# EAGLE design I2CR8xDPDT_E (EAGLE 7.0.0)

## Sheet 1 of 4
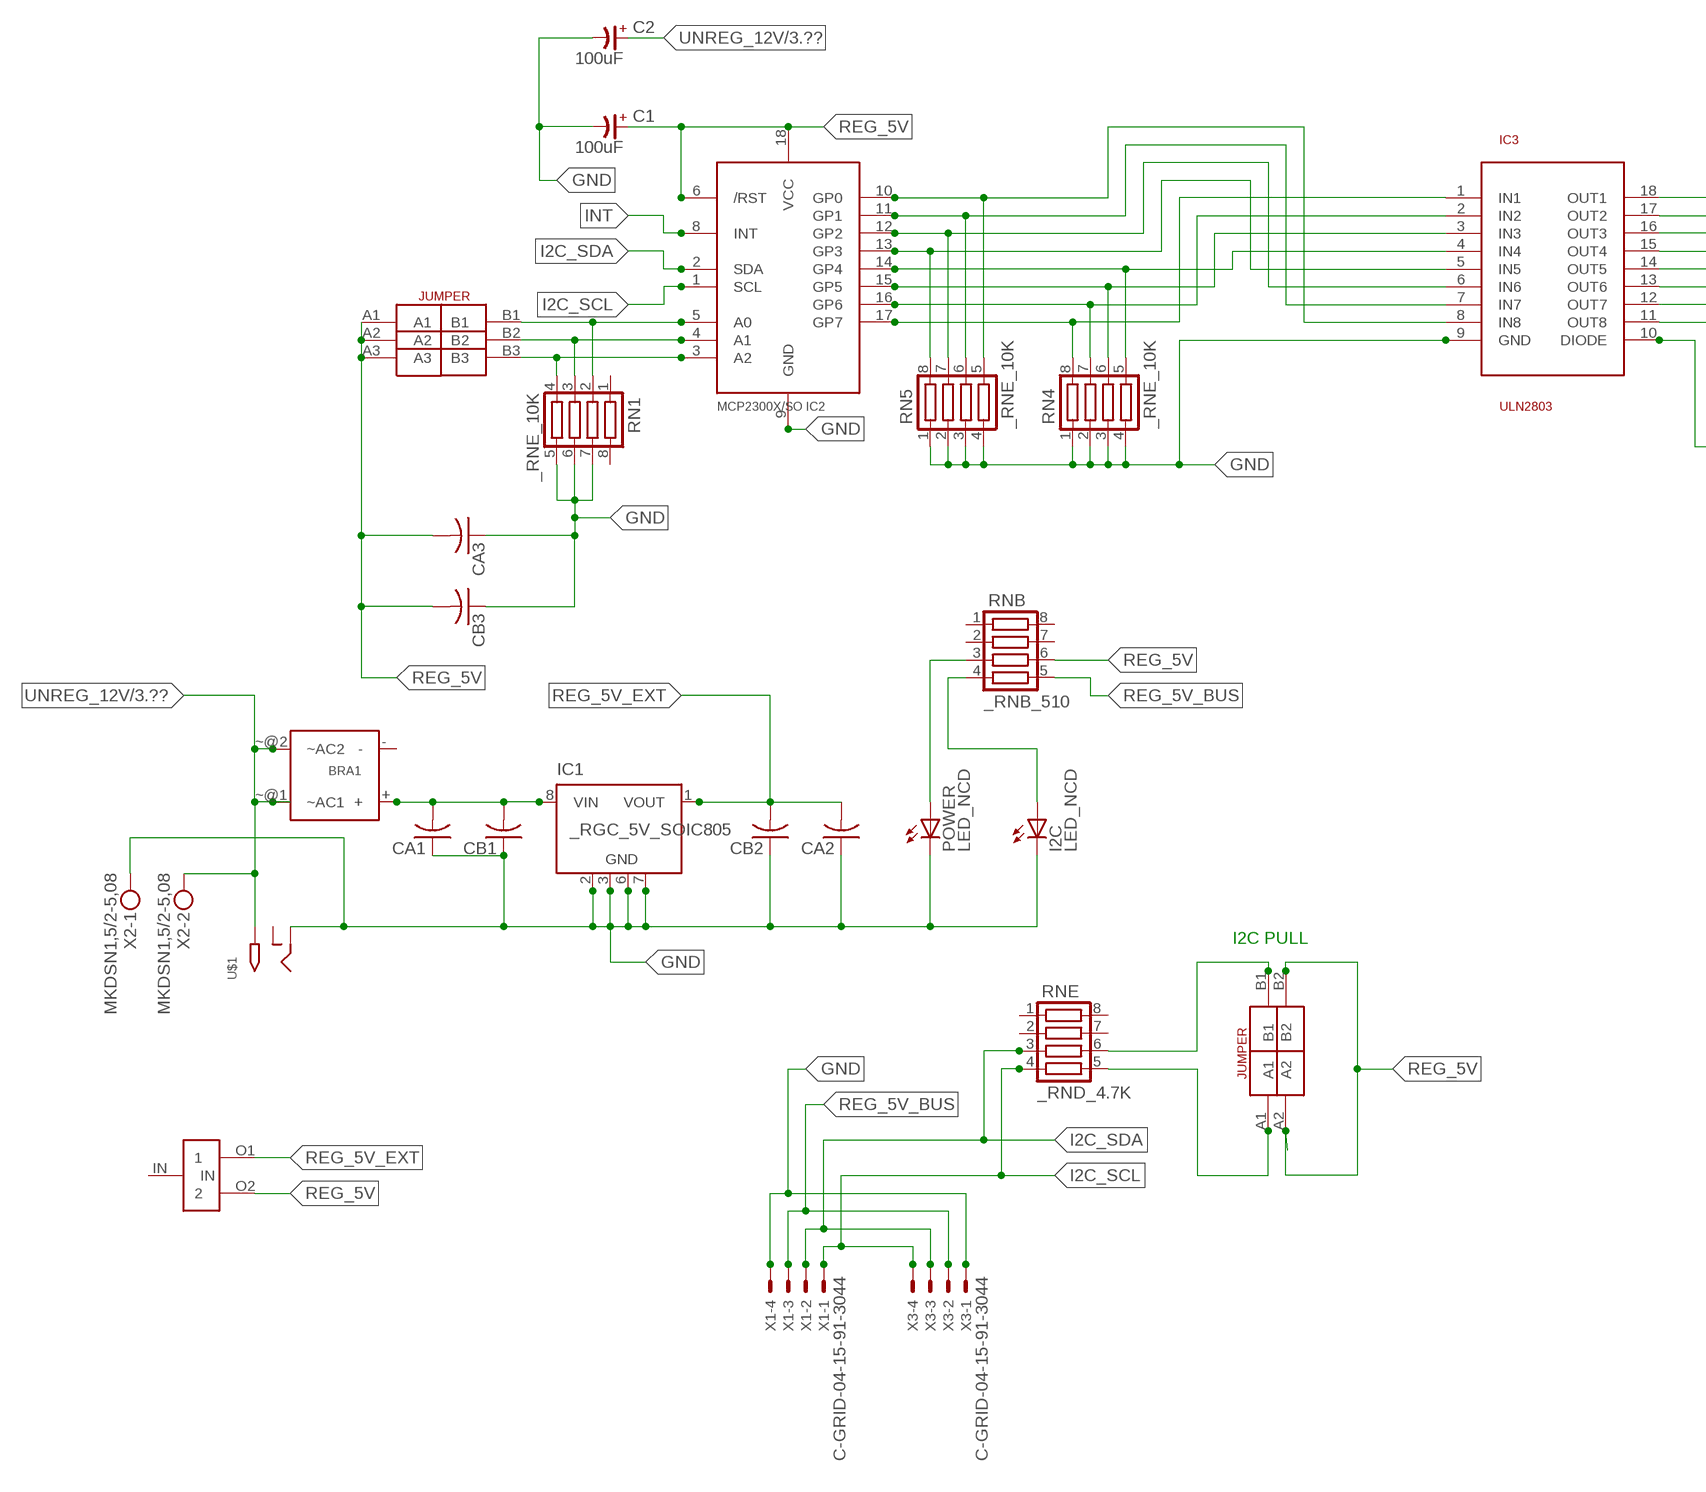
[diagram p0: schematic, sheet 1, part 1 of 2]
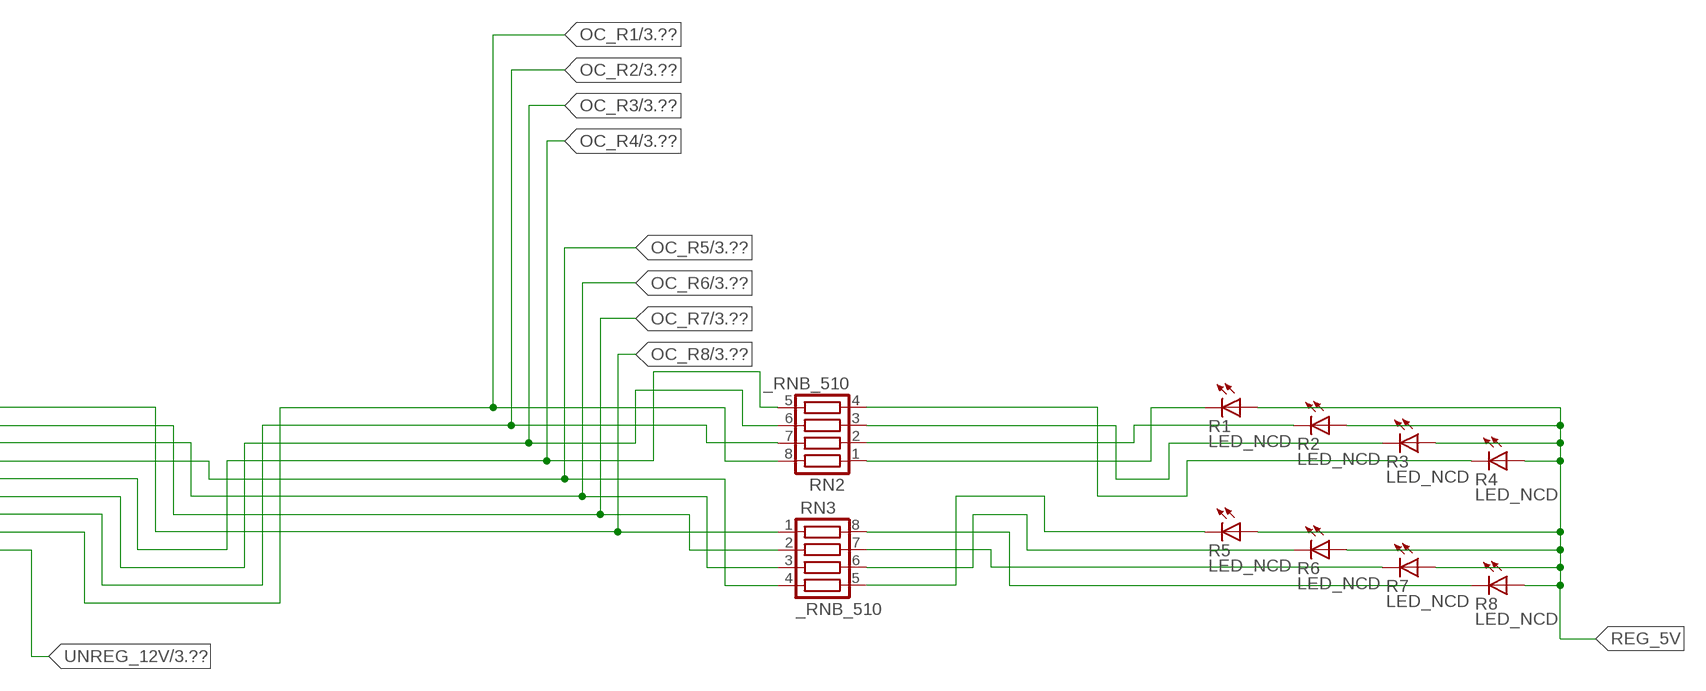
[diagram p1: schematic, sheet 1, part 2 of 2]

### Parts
BRA1  MB2S_  [MB2S]
C1  100uF  CP-E-025X060  [E-025X060]
C2  100uF  CP-E-025X060  [E-025X060]
CA1  CC1206KRX7R9BB104C1206K  [CC1206KRX7R9BB104]
CA2  CC1206KRX7R9BB104C1206K  [CC1206KRX7R9BB104]
CA3  CC1206KRX7R9BB104C1206K  [CC1206KRX7R9BB104]
CB1  TMK316F106ZL-TC1206K  [TMK316F106ZL-T]
CB2  TMK316F106ZL-TC1206K  [TMK316F106ZL-T]
CB3  TMK316F106ZL-TC1206K  [TMK316F106ZL-T]
I2C  LED_NCD  [CHIPLED_0603]
IC1  _RGC_5V_SOIC805  [_RGC_5V_SOIC8]
IC2  MCP2300X/SO  [SO18W]
IC3  ULN2803  [SO18L]
POWER  LED_NCD  [CHIPLED_0603]
R1  LED_NCD  [CHIPLED_0603]
R2  LED_NCD  [CHIPLED_0603]
R3  LED_NCD  [CHIPLED_0603]
R4  LED_NCD  [CHIPLED_0603]
R5  LED_NCD  [CHIPLED_0603]
R6  LED_NCD  [CHIPLED_0603]
R7  LED_NCD  [CHIPLED_0603]
R8  LED_NCD  [CHIPLED_0603]
RN1  _RNE_10K  [RNE]
RN2  _RNB_510  [RNB]
RN3  _RNB_510  [RNB]
RN4  _RNE_10K  [RNE]
RN5  _RNE_10K  [RNE]
RNB  _RNB_510  [RNB]
RNE  _RND_4.7K  [RND]
U$1  2.1MMJACK  [PJ-102A]
U$3  JUMPER_2X2  [JUMPER_2X2]
U$5  LINK_2  [LINK_2]
U$18  JUMPER_3X2  [JUMPER_3X2]
X1  C-GRID-04-15-91-3044  [15-91-04]
X2  MKDSN1,5/2-5,08  [MKDSN1,5/2-5,08]
X3  C-GRID-04-15-91-3044  [15-91-04]

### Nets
GND: C1.- C2.- CA1.1 CA2.1 CA3.1 CB1.1 CB2.1 CB3.1 I2C.C IC1.2(GND) IC1.3(GND) IC1.6(GND) IC1.7(GND) IC2.9(GND) IC3.9(GND) POWER.C RN1.5 RN1.6 RN1.7 RN4.1 RN4.2 RN4.3 RN4.4 RN5.1 RN5.2 RN5.3 RN5.4 U$1.RING X1.4 X2.1 X3.1
GP4: IC2.14(GP4) IC3.4(IN4) RN4.5
GP6: IC2.16(GP6) IC3.2(IN2) RN4.7
I2C_SCL: IC2.1(SCL) RNE.4 X1.1 X3.4
I2C_SDA: IC2.2(SDA) RNE.3 X1.2 X3.3
INT: IC2.8(INT)
N$1: BRA1.+ CA1.2 CB1.2 IC1.8(VIN)
N$2: POWER.A RNB.3
N$3: I2C.A RNB.4
N$4: RNE.5 U$3.A1
N$5: RNE.6 U$3.B1
N$6: IC2.5(A0) RN1.2 U$18.B1
N$7: IC2.4(A1) RN1.3 U$18.B2
N$8: IC2.3(A2) RN1.4 U$18.B3
N$20: R1.C RN2.1
N$21: IC2.12(GP2) IC3.6(IN6) RN5.7
N$22: IC2.11(GP1) IC3.7(IN7) RN5.6
N$23: IC2.10(GP0) IC3.8(IN8) RN5.5
N$29: R2.C RN2.2
N$30: R3.C RN2.3
N$31: R4.C RN2.4
N$32: R8.C RN3.8
N$81: R7.C RN3.7
N$82: R6.C RN3.6
N$83: R5.C RN3.5
N$89: IC2.13(GP3) IC3.5(IN5) RN5.8
N$93: IC2.15(GP5) IC3.3(IN3) RN4.6
N$94: IC2.17(GP7) IC3.1(IN1) RN4.8
OC_R1: IC3.11(OUT8) RN2.8 ; also sheet 3
OC_R2: IC3.12(OUT7) RN2.7 ; also sheet 3
OC_R3: IC3.13(OUT6) RN2.6 ; also sheet 3
OC_R4: IC3.14(OUT5) RN2.5 ; also sheet 3
OC_R5: IC3.15(OUT4) RN3.4 ; also sheet 3
OC_R6: IC3.16(OUT3) RN3.3 ; also sheet 3
OC_R7: IC3.17(OUT2) RN3.2 ; also sheet 3
OC_R8: IC3.18(OUT1) RN3.1 ; also sheet 3
REG_5V: C1.+ CA3.2 CB3.2 IC2.6(/RST) IC2.18(VCC) R1.A R2.A R3.A R4.A R5.A R6.A R7.A R8.A RNB.6 U$3.A2 U$3.B2 U$5.O2 U$18.A1 U$18.A2 U$18.A3
REG_5V_BUS: RNB.5 X1.3 X3.2
REG_5V_EXT: CA2.2 CB2.2 IC1.1(VOUT) U$5.O1
UNREG_12V: BRA1.~@1(~AC1) BRA1.~@2(~AC2) C2.+ IC3.10(DIODE) U$1.TIP X2.2 ; also sheet 3
Unconnected: BRA1.- IC1.4(NC) IC1.5(NC) RN1.1 RN1.8 RNB.1 RNB.2 RNB.7 RNB.8 RNE.1 RNE.2 RNE.7 RNE.8 U$1.RING_SW U$5.IN

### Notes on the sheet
- I2C PULL

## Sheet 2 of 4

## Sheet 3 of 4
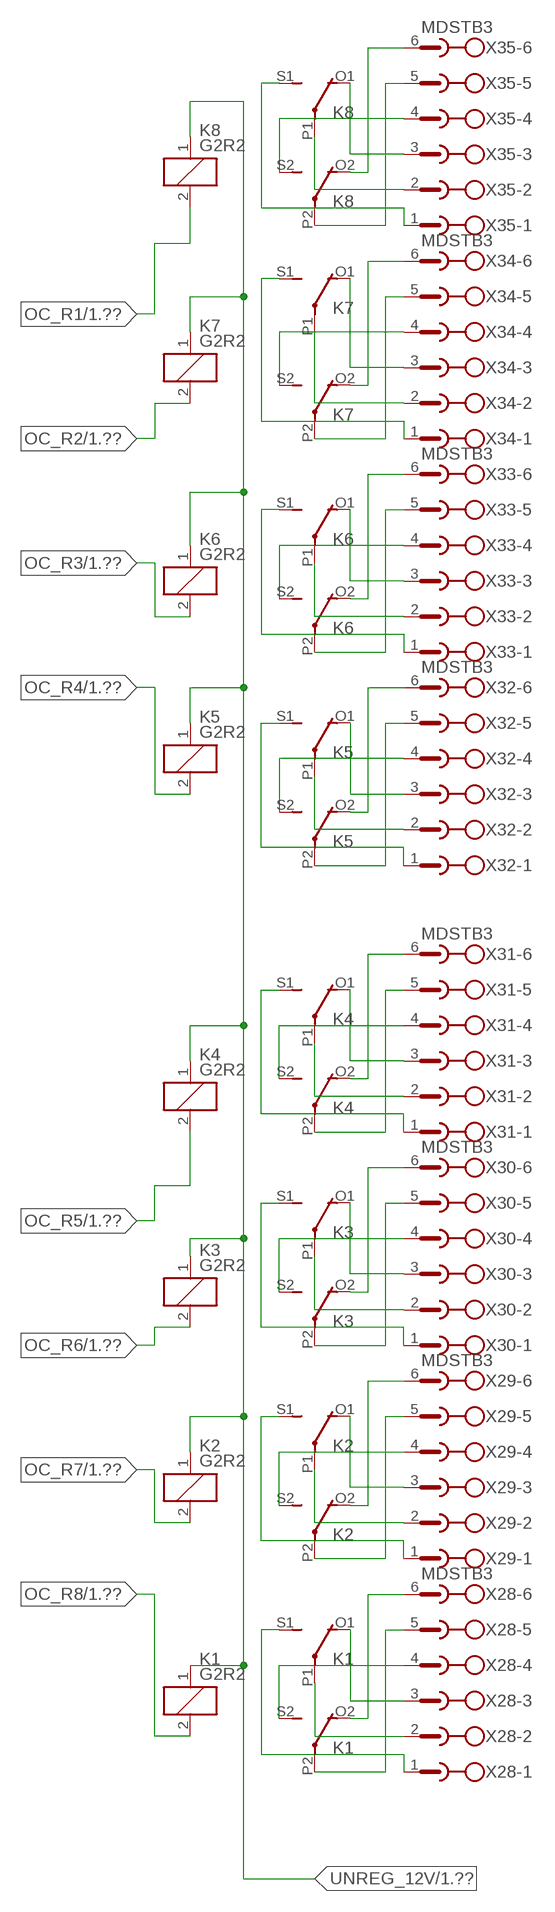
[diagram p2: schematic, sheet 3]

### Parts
K1  G2R2  [G2R2]
K2  G2R2  [G2R2]
K3  G2R2  [G2R2]
K4  G2R2  [G2R2]
K5  G2R2  [G2R2]
K6  G2R2  [G2R2]
K7  G2R2  [G2R2]
K8  G2R2  [G2R2]
X28  MDSTB3  [MDSTB3]
X29  MDSTB3  [MDSTB3]
X30  MDSTB3  [MDSTB3]
X31  MDSTB3  [MDSTB3]
X32  MDSTB3  [MDSTB3]
X33  MDSTB3  [MDSTB3]
X34  MDSTB3  [MDSTB3]
X35  MDSTB3  [MDSTB3]

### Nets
N$84: K1.P2(3:COM) X28.5
N$85: K1.O2(3:NC) X28.6
N$86: K1.S2(3:NO) X28.4
N$87: K1.P1(2:COM) X28.2
N$88: K1.O1(2:NC) X28.3
N$90: K1.S1(2:NO) X28.1
N$91: K2.P2(3:COM) X29.5
N$92: K2.O2(3:NC) X29.6
N$95: K2.S2(3:NO) X29.4
N$96: K2.S1(2:NO) X29.1
N$97: K2.P1(2:COM) X29.2
N$98: K2.O1(2:NC) X29.3
N$99: K3.P2(3:COM) X30.5
N$100: K3.O2(3:NC) X30.6
N$101: K4.P2(3:COM) X31.5
N$102: K4.O2(3:NC) X31.6
N$103: K3.S2(3:NO) X30.4
N$104: K4.S2(3:NO) X31.4
N$105: K3.O1(2:NC) X30.3
N$106: K4.O1(2:NC) X31.3
N$107: K4.P1(2:COM) X31.2
N$108: K3.P1(2:COM) X30.2
N$109: K3.S1(2:NO) X30.1
N$110: K4.S1(2:NO) X31.1
N$111: K5.O2(3:NC) X32.6
N$112: K5.P2(3:COM) X32.5
N$113: K5.S2(3:NO) X32.4
N$114: K5.P1(2:COM) X32.2
N$115: K5.S1(2:NO) X32.1
N$116: K5.O1(2:NC) X32.3
N$117: K6.P2(3:COM) X33.5
N$118: K6.O2(3:NC) X33.6
N$119: K6.P1(2:COM) X33.2
N$120: K6.S1(2:NO) X33.1
N$121: K7.P1(2:COM) X34.2
N$122: K8.P1(2:COM) X35.2
N$316: K8.P2(3:COM) X35.5
N$317: K8.O2(3:NC) X35.6
N$318: K6.O1(2:NC) X33.3
N$319: K8.O1(2:NC) X35.3
N$320: K7.O1(2:NC) X34.3
N$321: K7.O2(3:NC) X34.6
N$322: K7.P2(3:COM) X34.5
N$323: K6.S2(3:NO) X33.4
N$324: K7.S2(3:NO) X34.4
N$325: K7.S1(2:NO) X34.1
N$326: K8.S1(2:NO) X35.1
N$327: K8.S2(3:NO) X35.4
OC_R1: K8.2(1:C2) ; also sheet 1
OC_R2: K7.2(1:C2) ; also sheet 1
OC_R3: K6.2(1:C2) ; also sheet 1
OC_R4: K5.2(1:C2) ; also sheet 1
OC_R5: K4.2(1:C2) ; also sheet 1
OC_R6: K3.2(1:C2) ; also sheet 1
OC_R7: K2.2(1:C2) ; also sheet 1
OC_R8: K1.2(1:C2) ; also sheet 1
UNREG_12V: K1.1(1:C1) K2.1(1:C1) K3.1(1:C1) K4.1(1:C1) K5.1(1:C1) K6.1(1:C1) K7.1(1:C1) K8.1(1:C1) ; also sheet 1

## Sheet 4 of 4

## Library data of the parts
BRA1 = NCD_ULTIMATE_LIBRARY:MB2S: Bridge Rectifier BRA MB2S 200V 500ma Digikey MB2S-TPMSTR-ND/MB2S-TP
C1 C2 = NCD_ULTIMATE_LIBRARY:CP-: Capacitors All Kinds POLARIZED CAP
CA1-CA3 = NCD_ULTIMATE_LIBRARY:CC1206KRX7R9BB104: Capacitor CA .1uF 50V SMT C1206K CC1206KRX7R9BB104
CB1-CB3 = NCD_ULTIMATE_LIBRARY:TMK316F106ZL-T: Capacitor CB 10uF SMT 1206 TMK316F106ZL-T
I2C POWER = NCD_ULTIMATE_bhaskar:LED_NCD
IC1 = NCD_ULTIMATE_LIBRARY:_RGC_5V_SOIC8: Regulator Linear 5V Chip Positive VOLTAGE REGULATOR Digikey 497-7267-2-ND/L78L05CD13TR
IC2 = NCD_ULTIMATE_LIBRARY:MCP2300X: Semiconductor Port Expander I/O 8-Bit I2C MCP23008 Inexpensive i2c i/o expander - 8 general purpose i/o pins with optional pullups
IC3 = NCD_ULTIMATE_LIBRARY:ULN2803: Semiconductor 8 O.C. N-Channel Transistor Driver Digikey ULN2803AFWGCELTR-ND/ULN2803AFWG,C,EL
K1-K8 = NCD_ULTIMATE_LIBRARY:G2R2: RELAY 2 x switch, Omron
R1-R8 = NCD_ULTIMATE_LIBRARY:LED_NCD: LED Digikey 754-1132-2-ND/APT2012SRCPRV
RN1 RN4 RN5 = NCD_ULTIMATE_LIBRARY:_RNE_10K: Resistor Array RNE SMT 10K x 4 Single Resistor Source: http://www.ctscorp.com/components/Datasheets/CTSChipArrayDs.pdf Digikey 742C083103JPTR-ND/742C083103JP; OC_FARNELL: unknown; OC_NEWARK: unknown
RN2 RN3 RNB = NCD_ULTIMATE_LIBRARY:_RNB_510: Resistor Array RNB SMT 510 x 4 Single Resistor Source: http://www.ctscorp.com/components/Datasheets/CTSChipArrayDs.pdf Digikey 742C083511JPTR-ND/ 742C083511JP; OC_FARNELL: unknown; OC_NEWARK: unknown
RNE = NCD_ULTIMATE_LIBRARY:_RND_4.7K: Resistor Array RND SMT 4.7K x 4 Single Resistor Source: http://www.ctscorp.com/components/Datasheets/CTSChipArrayDs.pdf Digikey 742C083472JPTR-ND/742C083472JP; OC_FARNELL: unknown; OC_NEWARK: unknown
U$1 = NCD_ULTIMATE_CONNECTORS:2.1MMJACK: 2.1mm x 5.5mm DC jack with internal switch. Digikey part #PJ-102A, 4UCON part #05537 By microbuilder.eu
U$3 = NCD_ULTIMATE_CONNECTORS:JUMPER_2X2
U$5 = NCD_ULTIMATE_LIBRARY:LINK_2: PAD_top
U$18 = NCD_ULTIMATE_CONNECTORS:JUMPER_3X2
X1 X3 = NCD_ULTIMATE_CONNECTORS:C-GRID-04: CONNECTOR 4-Pos I2C wire to board 2.54 mm (0.100") pitch header Digikey WM1342-ND/0015912045; OC_FARNELL: unknown; OC_NEWARK: unknown
X2 = NCD_ULTIMATE_CONNECTORS:MKDSN1,5/2-5,08: MKDSN 1,5/ 2-5,08 Printklemme
X28-X35 = NCD_ULTIMATE_LIBRARY:MDSTB3: PHOENIX

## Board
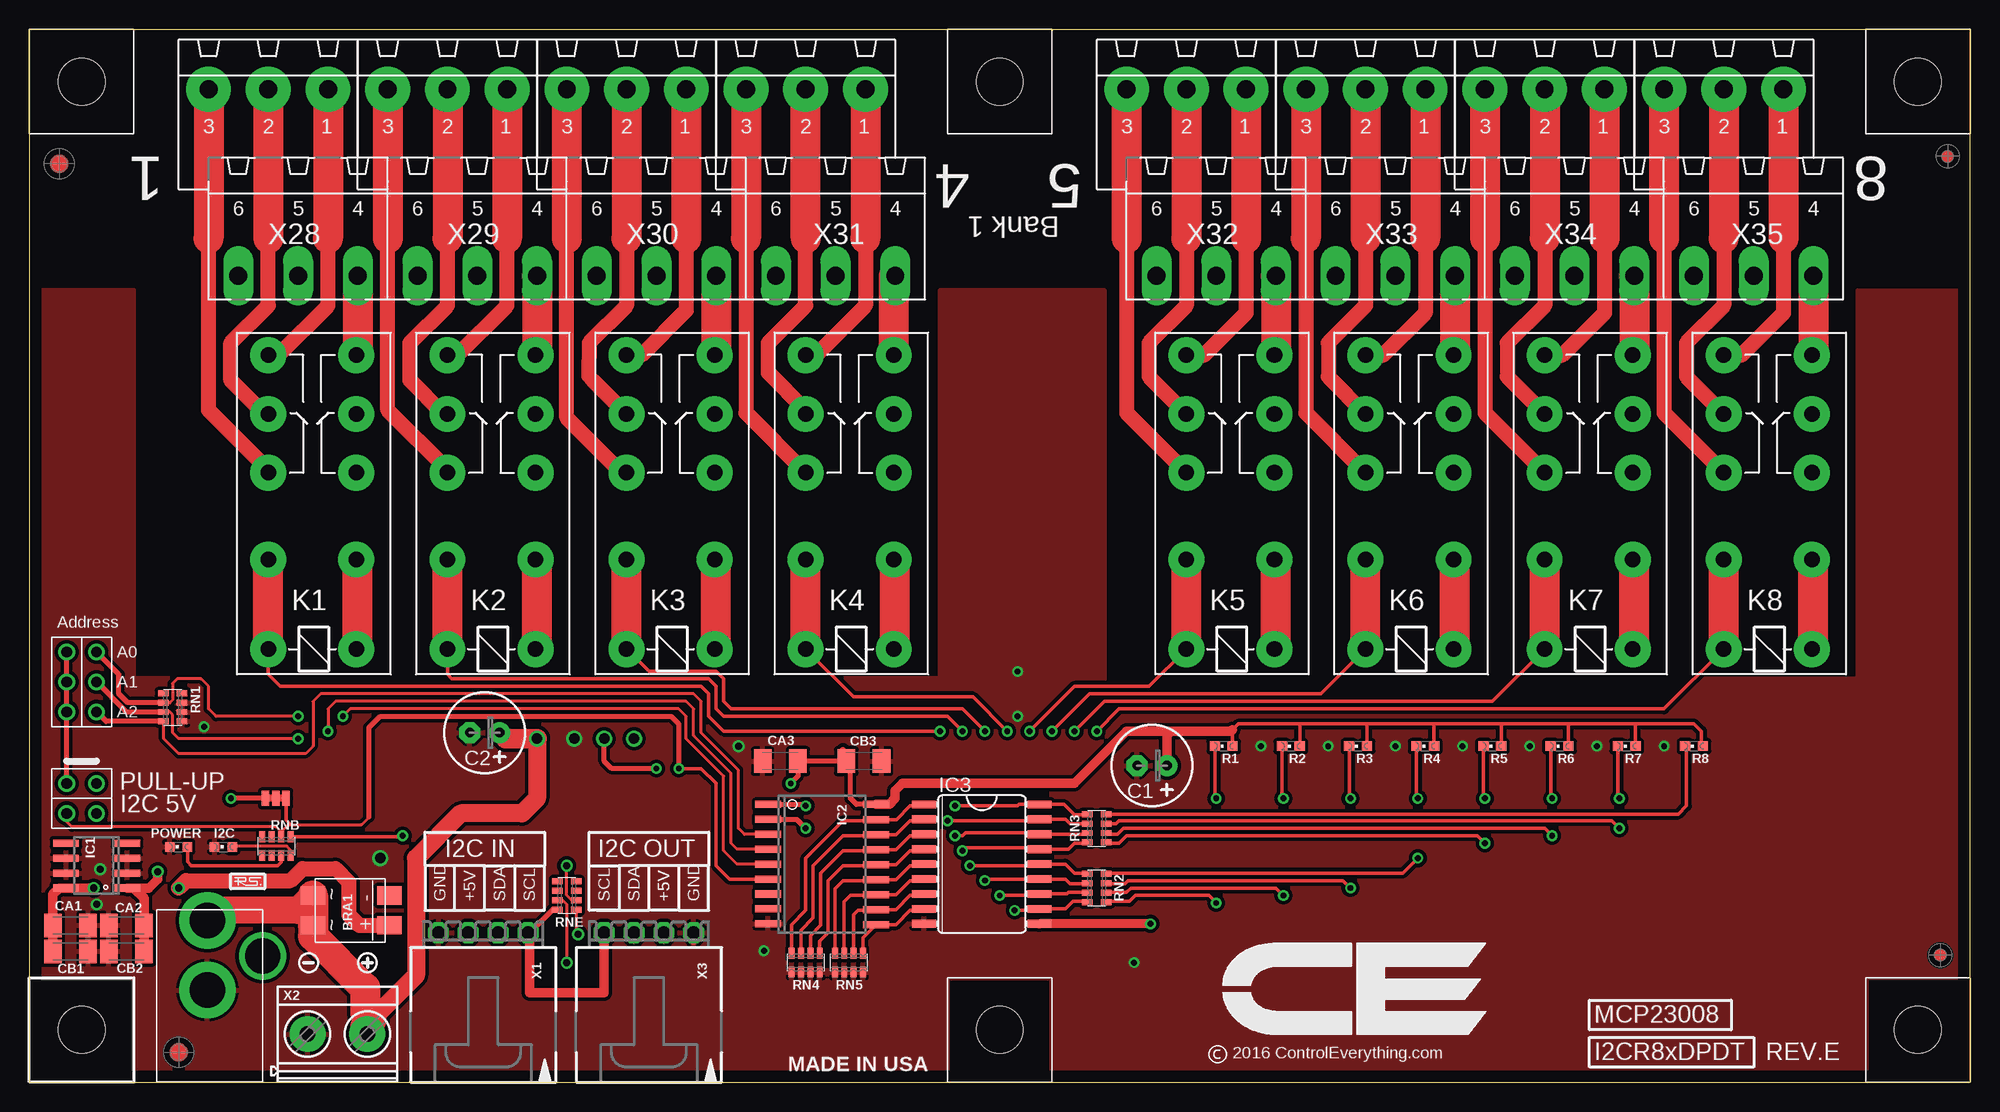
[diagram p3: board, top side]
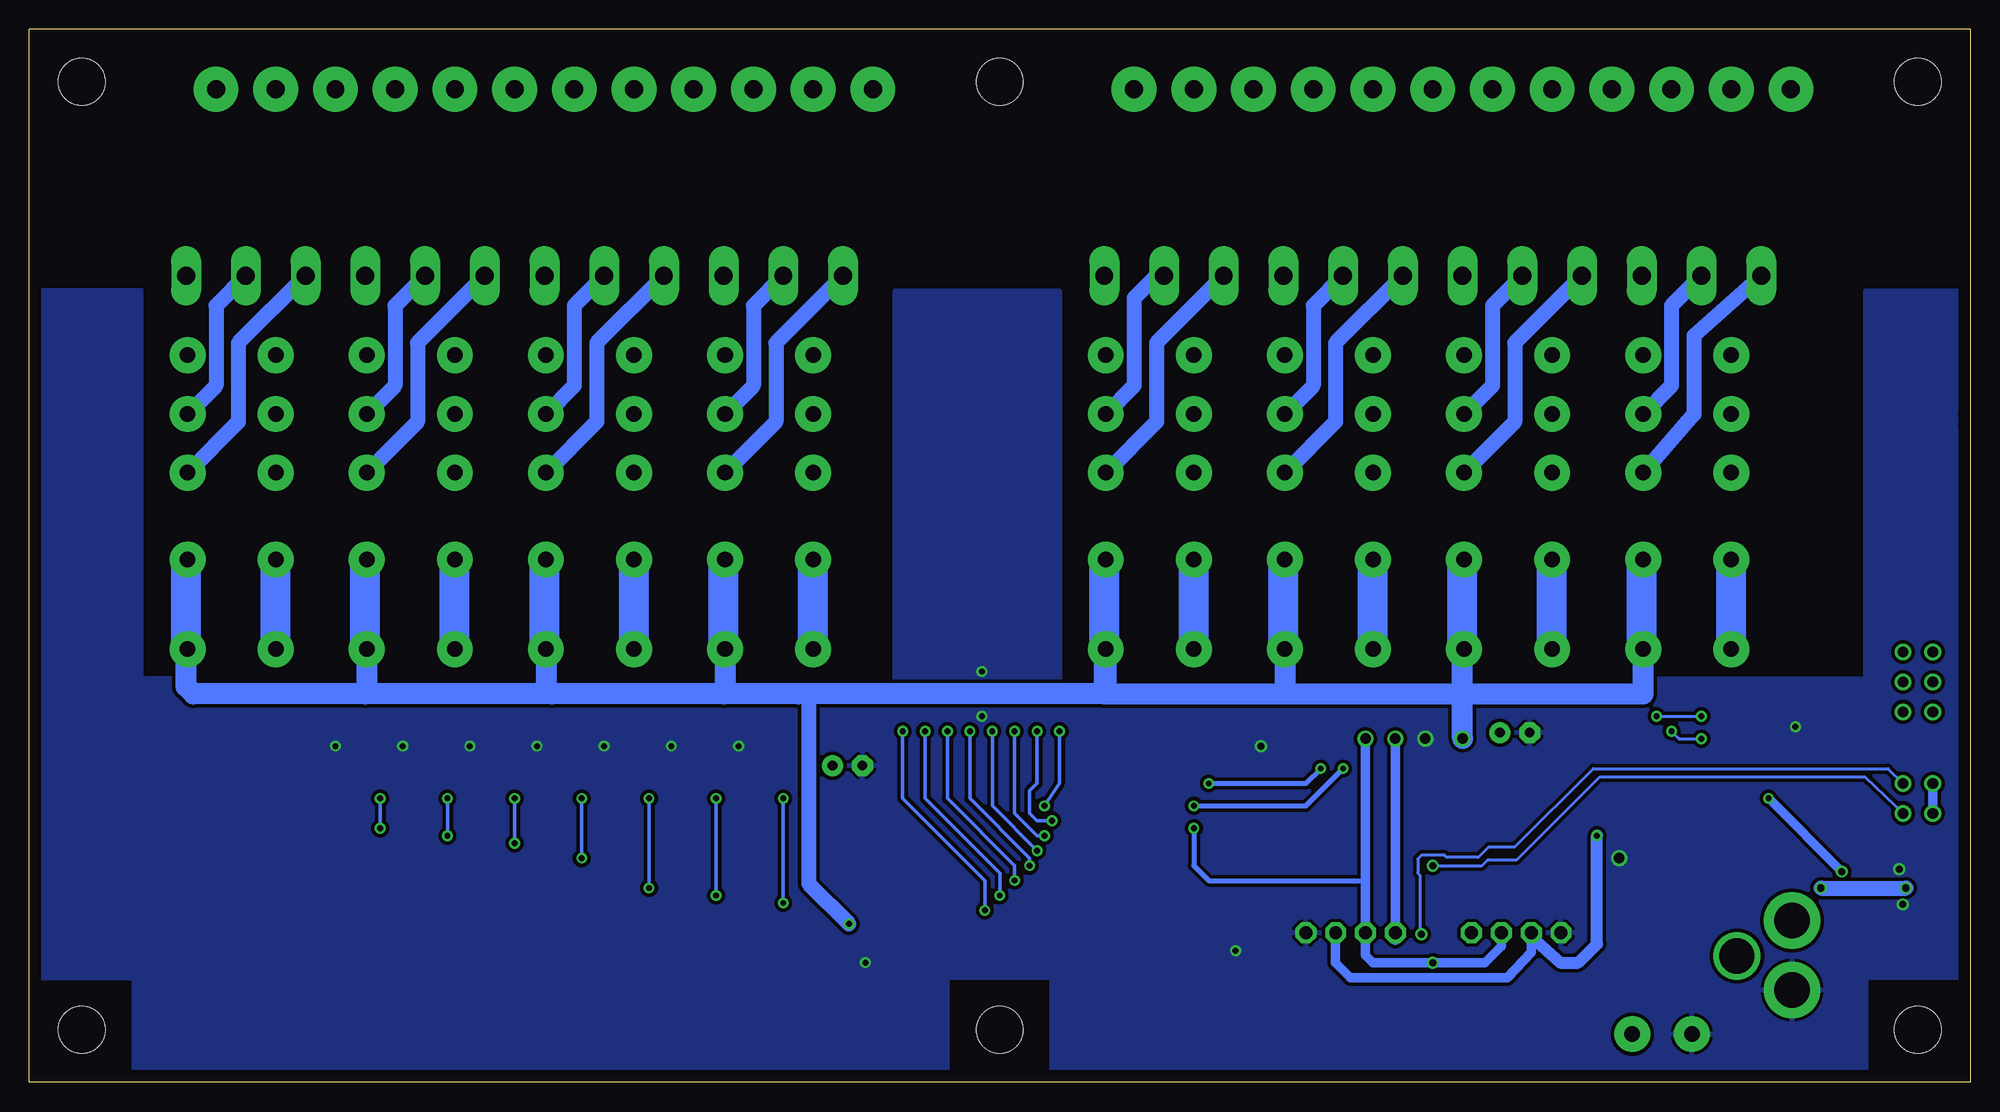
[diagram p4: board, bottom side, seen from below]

Size 165.1 x 89.53 mm. Coordinates in mm from the lower left corner, seen from the top.
Outline: 81.28,0 0,0 0,55.88
Outline: 81.28,0 82.53,0
Outline: 0,56.82 0,55.88
Outline: 81.28,0 165.1,0 165.1,89.53 0,89.53 0,55.88
Copper layers (1*16): Top 0.035mm / dielectric 1.5mm / Bottom 0.035mm
Design rules "default": minimum track width 10mil, minimum drill 24mil, track to track 8mil, track to pad 8mil, pad to pad 8mil, via to via 8mil, smd to smd 8mil, copper to edge 40mil, drill to drill 8mil, minimum pad ring 10mil, minimum via ring 8mil, stop-mask expansion 4mil, vias tented up to drill 0mil, thermal gap 10mil
Holes 3.96 mm at 4.45,4.45

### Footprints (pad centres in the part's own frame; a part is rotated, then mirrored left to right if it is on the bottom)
MB2S = smd 1.55 x 2.1: + 0,-6.5; - 2.54,-6.5; ~@1 0,0; ~@2 2.54,0
E-025X060 = drill 0.813 pad 1.778: + -1.27,0 | drill 0.813 pad 1.778 octagon: - 1.27,0
CC1206KRX7R9BB104 = smd 1.5 x 2: 1 -1.5,0; 2 1.5,0
TMK316F106ZL-T = smd 1.5 x 2: 1 -1.5,0; 2 1.5,0
CHIPLED_0603 = smd 0.8 x 0.8: A 0,-0.75; C 0,0.75
_RGC_5V_SOIC8 = smd 0.6 x 2.2: 1 -1.905,-2.6; 2 -0.635,-2.6; 3 0.635,-2.6; 4 1.905,-2.6; 5 1.905,2.6; 6 0.635,2.6; 7 -0.635,2.6; 8 -1.905,2.6
SO18W = smd 0.6 x 2.2: 1 -4.445,-4.6; 2 -3.175,-4.6; 3 -1.905,-4.6; 4 -0.635,-4.6; 5 0.635,-4.6; 6 1.905,-4.6; 7 3.175,-4.6; 8 4.445,-4.6; 9 5.715,-4.6; 10 5.775,4.6; 11 4.505,4.6; 12 3.235,4.6; 13 1.965,4.6; 14 0.695,4.6; 15 -0.575,4.6; 16 -1.845,4.6; 17 -3.145,4.6; 18 -4.445,4.6
SO18L = smd 0.66 x 2.032: 1 -5.08,-4.902; 2 -3.81,-4.902; 3 -2.54,-4.902; 4 -1.27,-4.902; 5 0,-4.902; 6 1.27,-4.902; 7 2.54,-4.902; 8 3.81,-4.902; 9 5.08,-4.902; 10 5.08,4.902; 11 3.81,4.902; 12 2.54,4.902; 13 1.27,4.902; 14 0,4.902; 15 -1.27,4.902; 16 -2.54,4.902; 17 -3.81,4.902; 18 -5.08,4.902
G2R2 = drill 1.321 pad 3.048: 1 -2.54,-3.683; 2 -2.54,3.81; 3 5.08,-3.683; 4 5.08,3.81; O1 12.471,3.81; O2 12.471,-3.683; P1 17.45,3.81; P2 17.45,-3.683; S1 22.454,3.81; S2 22.454,-3.683
CHIPLED_0603' = smd 0.8 x 0.876: A 0,-0.75; C 0,0.75
RNE = smd 0.5 x 0.9: 1 -1.2,-0.8; 2 -0.4,-0.8; 3 0.4,-0.8; 4 1.2,-0.8; 5 1.2,0.8; 6 0.4,0.8; 7 -0.4,0.8; 8 -1.2,0.8
RNB = smd 0.5 x 0.9: 1 -1.2,-0.8; 2 -0.4,-0.8; 3 0.4,-0.8; 4 1.2,-0.8; 5 1.2,0.8; 6 0.4,0.8; 7 -0.4,0.8; 8 -1.2,0.8
RND = smd 0.5 x 0.9: 1 -1.2,-0.8; 2 -0.4,-0.8; 3 0.4,-0.8; 4 1.2,-0.8; 5 1.2,0.8; 6 0.4,0.8; 7 -0.4,0.8; 8 -1.2,0.8
PJ-102A = drill 3 pad 4.8: RING 0.1,-3.39; TIP 0.1,-9.29 | drill 3 pad 3.251: RING_SW -4.6,-6.29
JUMPER_2X2 = drill 0.9: A1 0,2.54; A2 0,0; B1 2.54,2.54; B2 2.54,0
LINK_2 = smd 1.27 x 0.635: IN 0,0; O1 0,0.889; O2 0,-0.889
PCB_MOUNTING_HOLE = hole 3.962: 4.445,4.445
JUMPER_3X2 = drill 0.9: A1 0,5.08; A2 0,2.54; A3 0,0; B1 2.54,5.08; B2 2.54,2.54; B3 2.54,0
15-91-04 = drill 1.1 pad 1.778 octagon: 1 -3.81,-7.62; 2 -1.27,-7.62; 3 1.27,-7.62; 4 3.81,-7.62
MKDSN1,5/2-5,08 = drill 1.3 pad 3.048: 1 -2.561,0.025; 2 2.519,0.025
MDSTB3 = drill 1.524 pad 3.81: 1 -3.81,-10.795; 2 1.27,-10.795; 3 6.35,-10.795 | drill 1.524 pad 2.54 long: 4 -6.35,5.08; 5 -1.27,5.08; 6 3.81,5.08

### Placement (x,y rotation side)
BRA1  24.13,13.34 90 top
C1  95.5,26.92 180 top
C2  38.73,29.72 180 top
CA1  3.49,13.34 180 top
CA2  8.26,13.34 0 top
CA3  63.88,27.3 0 top
CB1  3.49,11.11 180 top
CB2  8.26,11.11 0 top
CB3  70.99,27.3 180 top
I2C  16.51,20 90 top
IC1  5.71,18.41 90 top
IC2  67.44,19.18 270 top
IC3  81.03,18.54 270 top
K1  24.13,39.37 90 top
K2  39.37,39.37 90 top
K3  54.61,39.37 90 top
K4  69.85,39.37 90 top
K5  102.23,39.37 90 top
K6  117.47,39.37 90 top
K7  132.72,39.37 90 top
K8  147.96,39.37 90 top
POWER  12.7,20 90 top
R1  LED_NCD  [CHIPLED_0603']  101.6,28.57 90 top
R2  LED_NCD  [CHIPLED_0603']  107.31,28.57 90 top
R3  LED_NCD  [CHIPLED_0603']  113.03,28.57 90 top
R4  LED_NCD  [CHIPLED_0603']  118.75,28.57 90 top
R5  LED_NCD  [CHIPLED_0603']  124.46,28.57 90 top
R6  LED_NCD  [CHIPLED_0603']  130.18,28.57 90 top
R7  LED_NCD  [CHIPLED_0603']  135.89,28.57 90 top
R8  LED_NCD  [CHIPLED_0603']  141.6,28.57 90 top
RN1  12.19,31.88 270 top
RN2  90.81,16.51 90 top
RN3  90.81,21.59 270 top
RN4  66.04,10.16 0 top
RN5  69.72,10.16 0 top
RNB  21.02,20.07 0 top
RNE  45.72,15.88 270 top
U$1  15.24,4.45 180 top
U$3  3.17,25.4 270 top
U$4  [VISION_REF10]  162.56,10.79 270 top
U$5  20.95,24.13 90 top
U$6  PCB_MOUNTING_HOLE  [PCB_MOUNTING_HOLE]  87,0 90 top
U$9  PCB_MOUNTING_HOLE  [PCB_MOUNTING_HOLE]  87,80.64 90 top
U$10  [VISION_REF15]  12.7,2.54 0 top
U$11  PCB_MOUNTING_HOLE  [PCB_MOUNTING_HOLE]  165.1,0 90 top
U$13  PCB_MOUNTING_HOLE  [PCB_MOUNTING_HOLE]  8.89,80.64 90 top
U$14  PCB_MOUNTING_HOLE  [PCB_MOUNTING_HOLE]  165.1,80.64 90 top
U$16  [VISION_REF10]  163.19,78.74 270 top
U$17  [VISION_REF15]  2.54,78.11 270 top
U$18  3.17,31.5 0 top
U$21  [ICON_USA]  64.52,0.89 0 top
U$22  [ICON_MINUS]  23.75,10.16 180 top
U$24  [ICON_PLUS]  28.77,10.16 90 top
X1  38.61,5.08 180 top
X2  26.23,4.06 0 top
X3  52.7,5.08 180 top
X28  21.59,73.66 180 top
X29  36.83,73.66 180 top
X30  52.07,73.66 180 top
X31  67.31,73.66 180 top
X32  99.69,73.66 180 top
X33  114.94,73.66 180 top
X34  130.18,73.66 180 top
X35  145.41,73.66 180 top

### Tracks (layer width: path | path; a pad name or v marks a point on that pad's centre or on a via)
GND  (via drill 0.5, 0.6, 0.9)
  Top 0.406: 34.8,12.38 X1.4
  Top 0.813: X3.1 56.52,12.06
  other vias: 5.71,15.11 6.03,18.1 46.35,29.21 29.84,19.05 14.86,30.23 62.48,11.18 127.64,28.57 93.98,10.16 133.35,28.57 139.06,28.57 121.92,28.57 116.2,28.57 110.49,28.57 104.78,28.57 60.33,28.57 84.07,31.11 84.07,34.92
  pour Bottom (isolate 0.305): 0.64,8.89 8.89,8.89 8.89,0 78.11,0 78.11,8.89 91.44,8.89 91.44,67.31 77.47,67.31 77.47,34.29 8.89,34.29 8.89,67.31 0.64,67.31
  pour Top (isolate 0.305): -1.27,8.89 8.89,8.89 8.89,0 78.11,0 78.11,8.89 91.44,8.89 91.44,67.31 77.47,67.31 77.47,34.29 8.89,34.29 8.89,67.31 -1.27,67.31
  pour Top (isolate 0.305): 87,34.29 155.57,34.29 155.57,67.31 164.47,67.31 164.47,8.89 156.21,8.89 156.21,0 87,0
  pour Bottom (isolate 0.305): 87,0 87,34.29 155.57,34.29 155.57,67.31 164.47,67.31 164.47,8.89 156.21,8.89 156.21,0
GP4
  Top 0.305: RN4.5 67.24,11.99 67.94,12.7 67.94,17.14 69.22,18.41 71.97,18.41 IC2.14 73.73,18.48 74.93,19.68 76,19.68 IC3.4
GP6
  Top 0.305: RN4.7 65.64,12.94 66.67,13.97 66.67,18.41 69.22,20.95 71.97,20.95 IC2.16 73.73,21.02 74.93,22.23 76,22.23 IC3.2
I2C_SCL  (via drill 0.5, 0.9)
  Top 0.406: RNE.4 44.51,14.68 42.55,12.7 | IC2.1 65.91,23.62 v66.04,23.5 | v53.34,26.67 49.53,26.67 48.9,27.3 v48.9,29.21
  Top 0.813: X3.4 48.9,7.62 42.55,7.62 42.55,12.7 X1.1
  Bottom 0.406: v66.04,23.5 56.52,23.5 v53.34,26.67
  Bottom 0.813: v48.9,29.21 X3.4 48.9,12.06
I2C_SDA  (via drill 0.5, 0.6, 0.9)
  Top 0.254: RNE.3 45.36,15.47 45.72,15.11 v45.72,10.16
  Top 0.406: IC2.2 65.28,22.35 v66.04,21.59
  Top 0.61: X3.3 51.44,12.06 | X1.2 39.88,12.38
  Bottom 0.406: v66.04,21.59 66.04,18.41 64.77,17.14 51.44,17.14 | 39.88,12.38 X1.2
  Bottom 0.813: 39.88,12.38 39.88,11.56 41.27,10.16 v45.72,10.16 50.8,10.16 51.44,10.79 X3.3 51.44,17.14 v51.44,29.21
N$1  (via drill 0.6)
  Top 0.813: CB1.2 CA1.2 1.99,15.96 2.54,16.51 IC1.8 v5.46,16.51
  Top 1.27: v12.7,16.51 13.34,17.14 22.23,17.14 23.24,18.16 26.04,18.16 27.18,17.02 27.18,14.22 28.07,13.34 BRA1.+
  Bottom 1.27: v12.7,16.51 v5.46,16.51
N$2
  Top 0.305: RNB.3 21.4,18.95 21.4,18.7 21.12,18.41 13.78,18.41 13.45,18.74 POWER.A
N$3
  Top 0.254: 22.23,18.95 22.23,19.74 21.9,20.07 16.94,20.07
  Top 0.305: RNB.4 22.23,18.95 | 16.94,20.07 I2C.A
N$4  (via drill 0.6)
  Top 0.254: RNE.5 46.52,12.6 v46.67,12.57
  Bottom 0.254: U$3.A1 6.99,26.67 32.07,26.67 38.73,20 40.96,20 41.85,19.11 44.51,19.11 44.7,19.3 46.67,19.3 46.99,18.99 46.99,17.78 46.8,17.59 46.8,12.7 v46.67,12.57
N$5  (via drill 0.6)
  Top 0.254: RNE.6 46.12,15.47 45.72,15.88 v45.72,18.41
  Bottom 0.254: v45.72,18.41 41.53,18.41 41.02,18.92 38.54,18.92 31.5,25.97 8.95,25.97 6.35,23.5 U$3.B1
N$6  (via drill 0.5)
  Top 0.254: IC2.5 60.2,18.54 59.05,19.68 59.05,26.04 55.88,29.21 55.88,31.11 55.24,31.75 27.3,31.75 v26.67,31.11 | v22.86,31.11 15.88,31.11 15.24,31.75 15.24,33.66 14.61,34.29 12.57,34.29 12.19,33.91 12.19,32.51 11.94,32.26 11.41,32.26 RN1.2
  Top 0.406: RN1.2 8.36,32.28 7.62,33.02 7.62,34.67 U$18.B1
  Bottom 0.254: v26.67,31.11 v22.86,31.11
N$7  (via drill 0.5)
  Top 0.254: IC2.4 60.2,19.81 59.69,20.32 59.69,26.29 56.52,29.46 56.52,31.75 55.88,32.38 26.04,32.38 25.4,31.75 v25.4,29.84 | v22.86,29.21 12.7,29.21 12.19,29.72 12.19,31.24 11.94,31.5 11.41,31.5 RN1.3
  Top 0.406: RN1.3 8.27,31.48 U$18.B2
  Bottom 0.254: v25.4,29.84 24.77,29.21 v22.86,29.21
N$8
  Top 0.254: IC2.3 60.83,21.08 60.33,21.59 60.33,26.54 57.15,29.72 57.15,32.38 56.52,33.02 24.77,33.02 24.13,32.38 24.13,28.57 23.5,27.94 12.7,27.94 11.43,29.21 11.43,30.64 RN1.4
  Top 0.406: RN1.4 6.53,30.68 U$18.B3
N$20  (via drill 0.5)
  Top 0.305: R1.C 100.85,24.25 v100.97,24.13 | v100.97,15.24 100.33,15.88 94.11,15.88 93.6,15.37 91.66,15.37 RN2.1
  Bottom 0.305: v100.97,24.13 v100.97,15.24
N$21
  Top 0.305: RN5.7 69.32,15.35 69.85,15.88 71.97,15.88 IC2.12 73.73,15.94 74.93,17.14 76,17.14 IC3.6
N$22
  Top 0.305: RN5.6 70.12,14.24 70.48,14.61 71.97,14.61 IC2.11 73.73,14.67 74.93,15.88 76,15.88 IC3.7
N$23
  Top 0.254: 71.97,13.34 IC2.10
  Top 0.305: RN5.5 70.92,12.29 IC2.10 73.73,13.4 74.93,14.61 76,14.61 IC3.8
N$29  (via drill 0.5)
  Top 0.305: R2.C 106.56,24.25 v106.68,24.13 | v106.68,15.88 106.05,16.51 93.73,16.51 93.34,16.13 91.62,16.13 RN2.2
  Bottom 0.305: v106.68,24.13 v106.68,15.88
N$30  (via drill 0.5)
  Top 0.305: R3.C 112.28,24.25 v112.39,24.13 | v112.39,16.51 111.76,17.14 93.47,17.14 93.22,16.89 91.62,16.89 RN2.3
  Bottom 0.305: v112.39,24.13 v112.39,16.51
N$31  (via drill 0.5)
  Top 0.305: R4.C 118,24.25 v118.11,24.13 | v118.11,19.05 116.84,17.78 91.67,17.78 RN2.4
  Bottom 0.305: v118.11,24.13 v118.11,19.05
N$32
  Top 0.305: RN3.8 140.26,22.79 140.97,23.5 140.97,28.46 R8.C
N$81  (via drill 0.5)
  Top 0.305: R7.C 135.14,24.25 v135.25,24.13 | v135.25,21.59 134.62,22.23 92.71,22.23 92.46,21.97 91.62,21.97 RN3.7
  Bottom 0.305: v135.25,24.13 v135.25,21.59
N$82  (via drill 0.5)
  Top 0.305: R6.C 129.43,24.25 v129.54,24.13 | v129.54,20.95 128.91,21.59 93.09,21.59 92.58,21.08 91.71,21.08 RN3.6
  Bottom 0.305: v129.54,24.13 v129.54,20.95
N$83  (via drill 0.5)
  Top 0.305: R5.C 123.71,24.25 v123.83,24.13 | v123.83,20.32 123.19,20.95 93.34,20.95 92.71,20.32 91.67,20.32 RN3.5
  Bottom 0.305: v123.83,24.13 v123.83,20.32
N$84
  Bottom 1.27: X28.5 25.4,66.04 25.4,59.23 K1.P2
N$85
  Bottom 1.27: X28.6 23.5,63.5 23.5,56.79 K1.O2
N$86
  Top 2.54: X28.4 27.94,61.95 K1.S2
N$87
  Top 1.27: K1.P1 20.02,56.82 17.14,59.69 17.14,62.87 20.32,66.04 20.32,71.75
  Top 2.54: X28.2 20.32,71.75
N$88
  Top 1.27: K1.O1 20.32,52.07 15.24,57.15 15.24,71.75
  Top 2.54: X28.3 15.24,71.75
N$89
  Top 0.305: RN5.8 68.52,16.45 69.22,17.14 71.97,17.14 IC2.13 73.73,17.21 74.93,18.41 76,18.41 IC3.5
N$90
  Top 1.27: K1.S1 21.18,61.82 25.4,66.04 25.4,71.75
  Top 2.54: X28.1 25.4,71.75
N$91
  Bottom 1.27: X29.5 40.64,66.04 40.64,59.23 K2.P2
N$92
  Bottom 1.27: X29.6 38.73,62.87 38.73,56.16 K2.O2
N$93
  Top 0.305: RN4.6 66.44,12.46 67.31,13.34 67.31,17.78 69.22,19.68 71.97,19.68 IC2.15 73.73,19.75 74.93,20.95 76,20.95 IC3.3
N$94
  Top 0.305: RN4.8 64.84,13.4 66.04,14.61 66.04,19.05 69.22,22.23 71.94,22.23 IC2.17 73.76,22.32 74.93,23.5 76,23.5 IC3.1
N$95
  Top 2.54: X29.4 43.18,61.95 K2.S2
N$96
  Top 1.27: K2.S1 36.32,61.72 40.64,66.04 40.64,71.75
  Top 2.54: X29.1 40.64,71.75
N$97
  Top 1.27: K2.P1 35.26,56.82 32.38,59.69 32.38,62.87 35.56,66.04 35.56,71.75
  Top 2.54: X29.2 35.56,71.75
N$98
  Top 1.27: K2.O1 35.56,52.07 30.48,57.15 30.48,71.75
  Top 2.54: X29.3 30.48,71.75
N$99
  Bottom 1.27: X30.5 55.88,66.04 55.88,59.23 K3.P2
N$100
  Bottom 1.27: X30.6 53.98,62.87 53.98,56.16 K3.O2
N$101
  Bottom 1.27: X31.5 69.22,68.58 71.12,66.67 71.12,59.23 K4.P2
N$102
  Bottom 1.27: X31.6 69.22,62.87 69.22,56.16 K4.O2
N$103
  Top 2.54: X30.4 58.42,61.95 K3.S2
N$104
  Top 2.54: X31.4 73.53,68.58 K4.S2
N$105
  Top 1.27: K3.O1 50.39,51.84 45.72,56.52 45.72,71.75
  Top 2.54: X30.3 45.72,71.75
N$106
  Top 1.27: 60.96,71.75 60.96,56.92 K4.O1
  Top 2.54: X31.3 60.96,71.75
N$107
  Top 1.27: K4.P1 66.04,57.15 62.87,60.33 62.87,62.87 66.04,66.04 66.04,71.75
  Top 2.54: 66.04,71.75 X31.2
N$108
  Top 1.27: 50.8,71.75 50.8,66.04 47.62,62.87 47.57,60.07 47.93,59.69 K3.P1
  Top 2.54: X30.2 50.8,71.75
N$109
  Top 1.27: 55.88,71.75 55.88,65.63 52.07,61.82 K3.S1
  Top 2.54: X30.1 55.88,71.75
N$110
  Top 1.27: 71.12,71.75 71.12,66.04 66.9,61.82 K4.S1
  Top 2.54: X31.1 71.12,71.75
N$111
  Bottom 1.27: X32.6 101.6,62.87 101.6,56.16 K5.O2
N$112
  Bottom 1.27: X32.5 103.5,66.04 103.5,59.23 K5.P2
N$113
  Top 2.54: X32.4 106.05,61.95 K5.S2
N$114
  Top 1.27: 98.42,71.75 98.42,66.04 95.25,62.87 95.25,59.99 K5.P1
  Top 2.54: X32.2 98.42,71.75
N$115
  Top 1.27: 103.5,71.75 103.5,65.41 99.92,61.82 K5.S1
  Top 2.54: X32.1 103.5,71.75
N$116
  Top 1.27: 93.34,71.75 93.34,56.92 K5.O1
  Top 2.54: X32.3 93.34,71.75
N$117
  Bottom 1.27: X33.5 118.75,66.04 118.75,59.23 K6.P2
N$118
  Bottom 1.27: X33.6 116.84,62.87 116.84,56.16 K6.O2
N$119
  Top 1.27: 113.67,71.75 113.67,66.04 110.49,62.87 110.49,59.99 K6.P1
  Top 2.54: X33.2 113.67,71.75
N$120
  Top 1.27: 118.75,71.75 118.75,65.41 115.16,61.82 K6.S1
  Top 2.54: X33.1 118.75,71.75
N$121
  Top 1.27: 128.91,71.75 128.91,66.04 125.73,62.87 125.73,59.99 K7.P1
  Top 2.54: X34.2 128.91,71.75
N$122
  Top 1.27: 144.15,71.75 144.15,66.04 140.97,62.87 140.97,59.99 K8.P1
  Top 2.54: X35.2 144.15,71.75
N$316
  Bottom 1.27: X35.5 149.22,66.04 149.22,59.23 K8.P2
N$317
  Bottom 1.27: X35.6 147.32,62.87 147.32,56.16 K8.O2
N$318
  Top 1.27: 108.58,71.75 108.58,56.92 K6.O1
  Top 2.54: X33.3 108.58,71.75
N$319
  Top 1.27: 139.06,71.75 139.06,56.92 K8.O1
  Top 2.54: X35.3 139.06,71.75
N$320
  Top 1.27: 123.83,71.75 123.83,56.92 K7.O1
  Top 2.54: X34.3 123.83,71.75
N$321
  Bottom 1.27: X34.6 132.08,62.87 132.08,56.16 K7.O2
N$322
  Bottom 1.27: X34.5 133.99,66.04 133.99,59.23 K7.P2
N$323
  Top 2.54: X33.4 121.28,61.95 K6.S2
N$324
  Top 2.54: X34.4 136.53,61.95 K7.S2
N$325
  Top 1.27: 133.99,71.75 133.99,65.41 130.4,61.82 K7.S1
  Top 2.54: X34.1 133.99,71.75
N$326
  Top 1.27: 149.22,71.75 149.22,65.41 145.64,61.82 K8.S1
  Top 2.54: X35.1 149.22,71.75
N$327
  Top 2.54: X35.4 151.76,61.95 K8.S2
OC_R1  (via drill 0.5)
  Top 0.305: RN2.8 89.95,15.37 88.77,15.37 88.14,14.73 IC3.11 85.8,14.61 v83.82,14.61 | K8.2 139.06,31.75 92.71,31.75 v90.81,29.84
  Bottom 0.305: v90.81,29.84 90.81,24.13 83.82,17.14 v83.82,14.61
OC_R2  (via drill 0.5)
  Top 0.305: RN2.7 89.99,16.13 88.39,16.13 88.27,16 IC3.12 85.8,15.88 v82.55,15.88 | v88.9,29.84 91.44,32.38 124.46,32.38 K7.2
  Bottom 0.305: v88.9,29.84 88.9,24.13 82.55,17.78 v82.55,15.88
OC_R3  (via drill 0.5)
  Top 0.305: RN2.6 89.99,16.89 88.52,16.89 88.14,17.27 IC3.13 81.53,17.27 81.41,17.14 v81.28,17.14 | K6.2 109.86,33.02 90.17,33.02 v87,29.84
  Bottom 0.305: v87,29.84 87,24.13 81.28,18.41 v81.28,17.14
OC_R4  (via drill 0.5)
  Top 0.305: RN2.5 89.94,17.78 88.9,17.78 88.14,18.54 IC3.14 85.8,18.41 v80.01,18.41 | v85.09,29.84 88.9,33.66 95.25,33.66 K5.2
  Bottom 0.305: v85.09,29.84 85.09,24.13 80.01,19.05 v80.01,18.41
OC_R5  (via drill 0.5)
  Top 0.305: RN3.4 89.94,20.32 88.9,20.32 88.39,19.81 IC3.15 85.8,19.94 79.63,19.94 v79.38,19.68 | v83.19,29.84 80.26,32.77 70.1,32.77 K4.2
  Bottom 0.305: v83.19,29.84 83.19,23.5 v79.38,19.68
OC_R6  (via drill 0.5)
  Top 0.305: RN3.3 89.9,21.08 IC3.16 85.8,21.21 79.63,21.21 79.38,20.95 v78.74,20.95 | v81.28,29.84 79.38,31.75 59.69,31.75 59.05,32.38 59.05,34.29 58.42,34.92 52.7,34.92 K3.2
  Bottom 0.305: v81.28,29.84 81.28,22.86 79.38,20.95 v78.74,20.95
OC_R7  (via drill 0.5)
  Top 0.305: RN3.2 89.99,21.97 88.52,21.97 88.14,22.35 IC3.17 85.8,22.23 v78.11,22.23 | v79.38,29.84 78.11,31.11 59.05,31.11 58.42,31.75 58.42,33.66 57.78,34.29 35.94,34.29 35.56,34.67 K2.2
  Bottom 0.305: v79.38,29.84 79.38,25.4 80.01,24.77 80.01,22.86 79.38,22.23 v78.11,22.23
OC_R8  (via drill 0.5)
  Top 0.305: RN3.1 89.95,22.73 88.9,22.73 88.01,23.62 IC3.18 84.2,23.62 84.07,23.5 v78.74,23.5 | v77.47,29.84 59.05,29.84 57.78,31.11 57.78,33.02 57.15,33.66 21.34,33.66 20.32,34.67 K1.2
  Bottom 0.305: v77.47,29.84 77.47,25.4 v78.74,23.5
REG_5V  (via drill 0.5)
  Top 0.254: RNB.6 21.42,21.29 | 21.42,21.29 22.04,21.91 22.23,21.91 28.26,21.91 28.89,22.54 | 21.42,21.29 20.99,21.72 3.62,21.72 3.17,22.16 U$3.B2
  Top 0.305: v55.24,26.67 57.15,26.67 58.42,25.4 58.42,18.41 59.56,17.27 IC2.6 | R1.A 102.35,29.96 102.87,30.48 107.95,30.48 | 107.95,30.48 113.67,30.48 | 113.67,30.48 119.38,30.48 | 119.38,30.48 125.09,30.48 | 125.09,30.48 130.81,30.48 | 130.81,30.48 136.53,30.48 | 136.53,30.48 141.6,30.48 142.24,29.84 142.24,28.69 R8.A | R7.A 136.64,30.36 136.53,30.48 | R6.A 130.93,30.36 130.81,30.48 | R5.A 125.21,30.36 125.09,30.48 | R4.A 119.5,30.36 119.38,30.48 | R3.A 113.78,30.36 113.67,30.48 | R2.A 108.06,30.36 107.95,30.48 | U$5.O2 21.84,22.29 22.23,21.91
  Top 0.406: U$18.A1 U$18.A2 U$18.A3 U$3.A2 | IC2.18 70.36,23.62 69.85,24.13 69.85,27.58 CB3.2 CA3.2 65.38,26.01 v64.77,25.4 | 62.71,17.14 IC2.6 | 28.89,22.54 28.89,30.16 29.84,31.11 54.61,31.11 55.24,30.48 v55.24,26.67
  Top 0.61: 69.22,28.22 CB3.2
  Top 0.813: IC2.18 73.15,23.62 73.66,24.13 73.66,24.77 74.3,25.4 88.9,25.4 93.34,29.84 97.16,29.84 | 97.16,29.84 102.23,29.84 102.35,29.96 | C1.+ 96.77,29.46 97.16,29.84
  Bottom 0.406: v64.77,25.4 56.52,25.4 v55.24,26.67
  Bottom 0.813: U$3.B2 U$3.A2
REG_5V_BUS  (via drill 0.5)
  Top 0.305: RNB.5 31.66,20.87 v31.75,20.95
  Top 0.61: X1.3 37.34,12.38 | X3.2 53.98,12.06
  Bottom 0.406: 37.34,12.38 X1.3 | 53.98,12.06 X3.2
  Bottom 0.813: 37.34,12.38 37.34,11.05 39.37,8.89 52.7,8.89 53.98,10.16 53.98,12.06
  Bottom 1.016: 37.34,12.38 34.86,10.16 33.34,10.16 31.75,11.75 v31.75,20.95
REG_5V_EXT  (via drill 0.5, 0.6)
  Top 0.406: U$5.O1 v17.14,24.13
  Top 0.813: CB2.2 CA2.2 9.76,15.64 8.89,16.51 | 8.89,16.51 IC1.1 | v10.92,17.91 10.92,17.27 10.16,16.51 8.89,16.51
  Bottom 0.813: v17.14,24.13 v10.92,17.91
UNREG_12V  (via drill 0.5, 0.9)
  Top 0.762: v95.38,13.46 IC3.10
  Top 1.524: v43.18,29.21 43.18,24.13 41.91,22.86 36.7,22.86 32.89,19.05 32.89,9.08 29.11,5.3 28.57,4.76
  Top 1.676: v43.18,29.21 40.51,29.21 C2.+
  Top 2.286: BRA1.~@2 22.86,14.61 16.01,14.61
  Top 2.54: 16.01,14.61 U$1.TIP | X2.2 28.55,4.45 28.57,4.76 | BRA1.~@2 BRA1.~@1 24.13,12.45 28.57,8 28.57,5.84 29.11,5.3
  Bottom 1.27: 98.81,33.02 98.81,16.89 v95.38,13.46
  Bottom 1.778: v43.18,29.21 43.18,33.02 | 43.18,33.02 27.81,33.02 K1.1 | 73.66,33.02 58.42,33.02 | 58.42,33.02 43.18,33.02 | 43.18,33.02 43.18,36.7 K2.1 | K3.1 58.29,33.15 58.42,33.02 | 106.05,33.02 99.69,33.02 98.81,33.02 73.66,33.02 | 106.05,33.02 120.65,33.02 | 120.65,33.02 136.53,33.02 | 136.53,33.02 151.13,33.02 151.76,33.66 151.76,36.7 K8.1 | K7.1 136.4,33.15 136.53,33.02 | K6.1 121.16,33.53 120.65,33.02 | K5.1 105.92,33.15 106.05,33.02 | 73.66,33.02 73.66,36.7 K4.1 73.53,33.15 73.66,33.02

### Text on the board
tNames: 1 | 8 | 4 | 5 | Bank 1 | Address | A0 | A1 | A2 | PULL-UP | I2C 5V | I2C IN | I2C OUT | GND | +5V | SDA | SCL | SCL | SDA | +5V | +5V | GND | MCP23008 | 2016 ControlEverything.com | I2CR8xDPDT | REV.E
